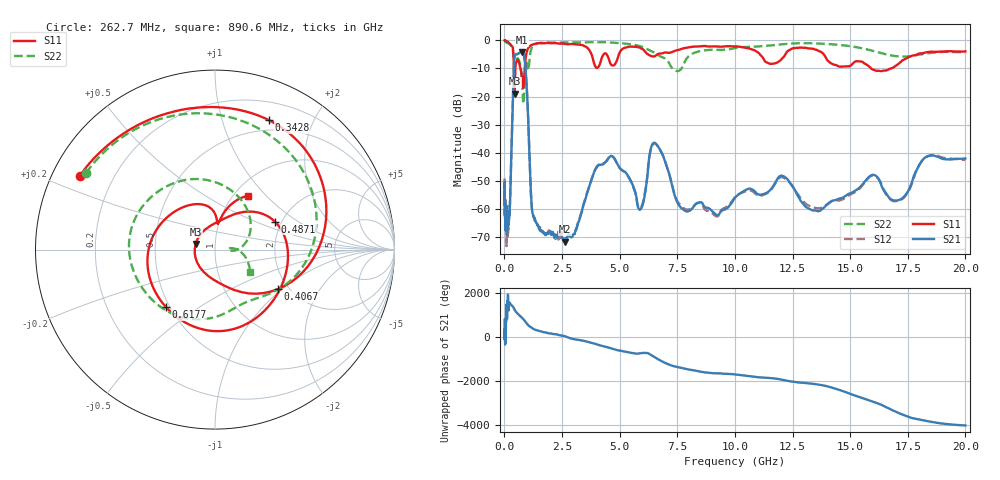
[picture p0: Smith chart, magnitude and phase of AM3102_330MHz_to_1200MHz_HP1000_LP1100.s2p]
! Date/Time: Tue, Sep 11, 2018 5:17 PM
! Network Analyzer: Agilent Technologies E8362B Rev: A.07.50.63
! Sweep from 0.010 to 20.000 GHz, 1601 Points, Sweep Type: LOG
! Power Supply: 4.949 V, 0.001 A
# Hz S DB R 50
!freq MagS11 AngS11 MagS21 AngS21 MagS12 AngS12 MagS22 AngS22
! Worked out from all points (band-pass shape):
!   1601 points, 10 MHz to 20 GHz, reference 50 ohm
!   highest |S21| = -4.16 dB at 754.2 MHz (marker M1); lowest = -71.7 dB at 2.631 GHz (marker M2)
!   |S21| within 3 dB of the highest: 425 MHz to 884.2 MHz (459.2 MHz wide, 70.1 % of centre)
!   lowest |S11| = -19.0 dB at 440.9 MHz (marker M3), VSWR 1.25, Z = 40.2 + j2.55 ohm
!   |S11| at or under -10 dB: 413.9 MHz to 474.7 MHz (60.83 MHz wide, 13.7 % of centre); 696.9 MHz to 881.3 MHz (184.4 MHz wide, 23.4 % of centre); 15.91 GHz to 16.77 GHz (860.9 MHz wide, 5.27 % of centre)
!   |S22| runs from -22.5 to -0.2 dB; largest |S21 - S12| = 0.01
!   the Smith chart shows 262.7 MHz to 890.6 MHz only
!   S11 on the Smith chart (normalised r, x): 262.7 MHz: 0.08, +0.25; 342.8 MHz: 0.38, +1.43; 406.7 MHz: 1.77, -0.94; 487.1 MHz: 1.85, +0.67; 617.7 MHz: 0.48, -0.37; 890.6 MHz: 1.16, +0.80
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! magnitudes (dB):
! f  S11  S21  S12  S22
! 10 MHz  0.0  -52.8  -49.2  -0.3
! 35.55 MHz  0.0  -62.6  -65.3  -0.5
! 126.4 MHz  -0.4  -64.0  -62.9  -0.9
! 262.7 MHz  -1.3  -53.1  -52.4  -1.6
! 342.8 MHz  -2.1  -28.3  -28.4  -2.7
! 406.7 MHz  -7.6  -10.1  -10.2  -6.3
! 440.9 MHz  -19.0  -5.8  -5.9  -9.3
! 447.2 MHz  -18.4  -5.5  -5.6  -9.4
! 487.1 MHz  -8.7  -5.1  -5.1  -7.8
! 617.7 MHz  -7.5  -4.5  -4.6  -6.8
! 754.2 MHz  -12.8  -4.2  -4.2  -13.1
! 890.6 MHz  -9.0  -7.6  -7.7  -12.7
! 1.196 GHz  -1.6  -60.1  -60.2  -2.4
! 1.59 GHz  -1.0  -67.9  -67.5  -0.9
! 2.631 GHz  -1.3  -71.7  -70.6  -0.7
! 4.543 GHz  -6.9  -41.7  -41.6  -0.7
! 5.652 GHz  -2.2  -53.4  -53.7  -1.6
! 6.549 GHz  -5.5  -36.6  -36.8  -4.6
! 7.697 GHz  -3.0  -60.0  -59.3  -9.8
! 9.047 GHz  -2.1  -61.2  -61.8  -3.3
! 17.02 GHz  -8.8  -57.1  -57.3  -5.6
! 20 GHz  -3.9  -42.1  -42.6  -4.2
